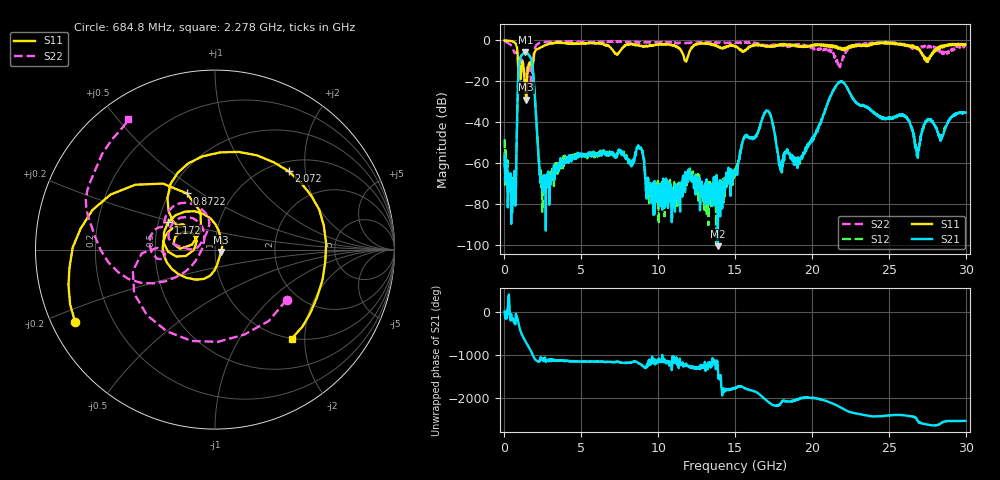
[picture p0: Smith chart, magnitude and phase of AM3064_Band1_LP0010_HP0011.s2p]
# Hz S DB R 50.0
!freq dBS11 angS11 dBS21 angS21 dBS12 angS12 dBS22 angS22
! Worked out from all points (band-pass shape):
!   1600 points, 10 MHz to 29.98 GHz, reference 50 ohm
!   highest |S21| = -5.70 dB at 1.36 GHz (marker M1); lowest = -100.4 dB at 13.88 GHz (marker M2)
!   |S21| within 3 dB of the highest: 1.027 GHz to 1.716 GHz (688.6 MHz wide, 50.2 % of centre)
!   lowest |S11| = -28.8 dB at 1.416 GHz (marker M3), VSWR 1.07, Z = 53.4 - j1.45 ohm
!   |S11| at or under -10 dB: 876.6 MHz to 1.877 GHz (1 GHz wide, 72.7 % of centre); 11.75 GHz to 11.84 GHz (92.18 MHz wide, 0.781 % of centre); 27.4132 GHz to 27.43835 GHz (25.14 MHz wide, 0.0917 % of centre)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
!   |S22| runs from -22.8 to -0.3 dB; largest |S21 - S12| = 0.0058
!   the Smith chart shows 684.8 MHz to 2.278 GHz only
!   S11 on the Smith chart (normalised r, x): 684.8 MHz: 0.07, -0.24; 872.2 MHz: 0.61, +0.44; 1.172 GHz: 0.56, +0.19; 2.072 GHz: 1.19, +1.62; 2.278 GHz: 1.00, -1.73
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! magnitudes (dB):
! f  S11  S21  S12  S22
! 10 MHz  0.0  -55.8  -48.3  -0.3
! 684.8 MHz  -1.1  -80.5  -75.5  -6.2
! 872.2 MHz  -9.1  -23.1  -23.1  -9.8
! 1.172 GHz  -10.4  -6.8  -6.7  -9.8
! 1.36 GHz  -24.1  -5.7  -5.7  -21.1
! 1.416 GHz  -28.8  -5.8  -5.8  -17.9
! 1.791 GHz  -13.0  -10.8  -10.8  -17.6
! 2.072 GHz  -4.4  -38.9  -39.2  -2.2
! 2.278 GHz  -3.7  -65.4  -61.2  -1.2
! 2.597 GHz  -2.5  -70.5  -69.1  -0.8
! 5.015 GHz  -1.4  -56.2  -56.7  -0.7
! 8.782 GHz  -2.7  -52.2  -52.7  -0.8
! 10 GHz  -2.0  -72.5  -75.1  -0.9
! 13.88 GHz  -3.1  -100.4  -75.1  -1.3
! 15 GHz  -2.9  -63.2  -65.6  -1.2
! 17.05 GHz  -2.9  -34.4  -34.2  -2.6
! 17.97 GHz  -2.4  -63.0  -63.2  -2.1
! 19.99 GHz  -2.8  -48.7  -48.2  -3.3
! 21.85 GHz  -3.5  -20.2  -20.1  -12.5
! 25 GHz  -1.0  -38.2  -38.2  -1.2
! 26.85 GHz  -4.3  -54.2  -55.1  -3.2
! 29.98 GHz  -1.9  -35.2  -35.1  -3.2
